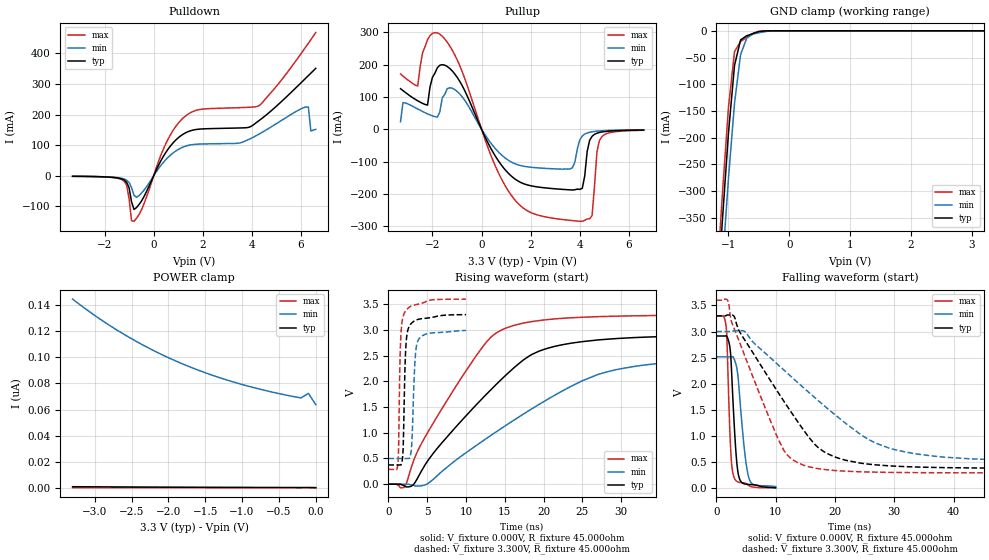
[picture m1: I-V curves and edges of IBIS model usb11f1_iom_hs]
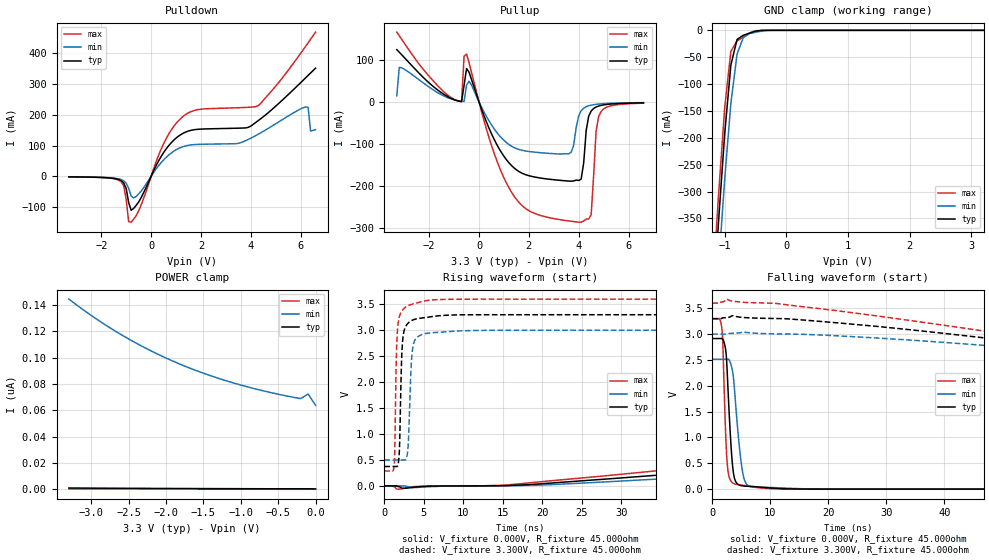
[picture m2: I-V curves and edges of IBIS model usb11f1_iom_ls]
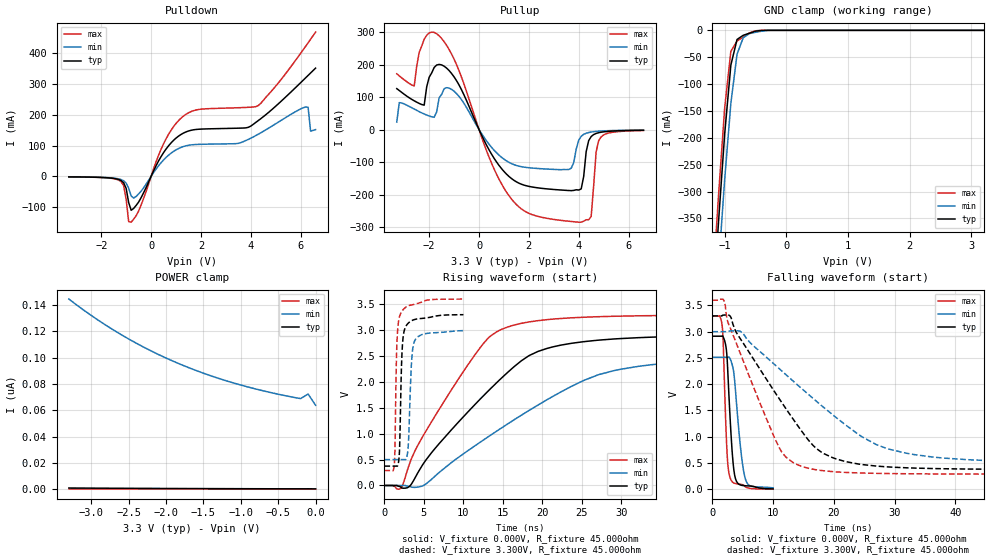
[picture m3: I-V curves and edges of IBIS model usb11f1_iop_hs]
[IBIS Ver]  4.0
[File Name]  lpc2939_lqfp208.ibs
[File Rev]  1.0
[Date]  Fri Feb 27 10:34:29 2009
[Source]  Package model is generic
[Notes]   IO models Rev 0.20 IBIS Model Design Automation Generation
[Copyright]  NXP Semiconductors 2009. All rights reserved.
[Disclaimer]
| NXP Semiconductors warrants and represents that the IBIS models
| identified herein are owned by NXP Semiconductors (NXP).  The
| models provided are not warranted as fully representing all of the
| operating characteristics and specifications of the semiconductor
| products to which the models relate.  Moreover, unless there is a
| signed, written agreement to the contrary, these models are furnished
| on an "as is" basis without support or warranty of any kind, either
| expressed or implied, regarding the use thereof, and NXP
| specifically disclaims all implied warranties of merchantability and
| fitness of the models for any purpose.
| NXP does not assume any liability arising out of the application
| or use of these IBIS models including infringement of patents and
| copyrights, nor does NXP convey any license under its patents and
| copyrights or the rights of others.
| NXP provides IBIS models as a service to our customers.  You and
| your company shall not distribute, convey, sell, or give these models
| to anyone else without receiving prior written permission from
| NXP.
[Component]   LPC23XX_LQFP208_01
[Manufacturer]  NXP
[Package]
|[Package Model]  LQFP208
|variable   typ   min   max
R_pkg   130.00m   123.00m   137.00m
L_pkg   8.30nH   7.50nH   9.20nH
C_pkg   1.00pF   0.80pF   1.30pF
| IMPORTANT NOTES:
| This model is valid for the following part types:
| LPC2939, LPC2930
| Signal names may be slightly different from the data
| sheet due to the 20 Char length limitation
[Pin]   signal_name   model_name   | comments
1 TDO bpats5thpept5v
2 P2_21 bpats5thpept5v
3 P0_24 bpats5thpept5v
4 P0_25 bpats5thpept5v
5 P0_26 bpats5thpept5v
6 P0_27 bpats5thpept5v
7 P0_28 bpats5thpept5v
8 P0_29 bpats5thpept5v
9 VDDE_10 POWER
10 P2_22 bpats5thpept5v
11 P2_23 bpats5thpept5v
12 P3_6 bpats5thpept5v
13 P3_7 bpats5thpept5v
14 P0_30 bpats5thpept5v
15 P0_31 bpats5thpept5v
16 P2_24 bpats5thpept5v
17 P2_25 bpats5thpept5v
18 GNDE_21 POWER
19 USB1_IOP usb11f1_iop_ls
20 USB1_IOM usb11f1_iom_ls
21 USB2_IOP usb11f1_iop_ls
22 USB2_IOM usb11f1_iom_ls
23 VDDE_26 POWER
24 VDD_27 POWER
25 GND_28 POWER
26 P1_31 bpats5thpept5v
27 GNDE_30 POWER
28 P4_0 bpats5thpept5v
29 P1_30 bpats5thpept5v
30 P5_0 bpats5thpept5v
31 P3_8 bpats5thpept5v
32 P3_9 bpats5thpept5v
33 P1_29 bpats5thpept5v
34 VDDE_37 POWER
35 P4_16 bpats5thpept5v
36 P1_28 bpats5thpept5v
37 P2_26 bpats5thpept5v
38 P4_8 bpats5thpept5v
39 GNDE_42 POWER
40 P2_27 bpats5thpept5v
41 P5_8 bpats5thpept5v
42 P1_27 bpats5thpept5v
43 P1_26 bpats5thpept5v
44 P4_20 bpats5thpept5v
45 VDDE_48 POWER
46 P1_25 bpats5thpept5v
47 GND_50 POWER
48 VDD_51 POWER
49 P1_24 bpats5thpept5v
50 P1_23 bpats5thpept5v
51 P1_22 bpats5thpept5v
52 TMS bpats5thpept5v
53 TCK bpats5thpept5v
54 P1_21 bpats5thpept5v
55 P1_20 bpats5thpept5v
56 P1_19 bpats5thpept5v
57 P1_18 bpats5thpept5v
58 P1_17 bpats5thpept5v
59 GNDE_62 POWER
60 P4_4 bpats5thpept5v
61 P1_16 bpats5thpept5v
62 P5_4 bpats5thpept5v
63 P2_0 bpats5thpept5v
64 P4_12 bpats5thpept5v
65 P2_1 bpats5thpept5v
66 P5_12 bpats5thpept5v
67 VDDE_70 POWER
68 P4_1 bpats5thpept5v
69 P3_10 bpats5thpept5v
70 GND_73 POWER
71 VDD_74 POWER
72 P5_1 bpats5thpept5v
73 P3_11 bpats5thpept5v
74 P4_17 bpats5thpept5v
75 P1_15 bpats5thpept5v
76 P4_9 bpats5thpept5v
77 GNDE_80 POWER
78 P5_9 bpats5thpept5v
79 P1_14 bpats5thpept5v
80 P4_21 bpats5thpept5v
81 P1_13 bpats5thpept5v
82 P4_5 bpats5thpept5v
83 P1_12 bpats5thpept5v
84 P5_5 bpats5thpept5v
85 VDDE_88 POWER
86 P2_2 bpats5thpept5v
87 P2_3 bpats5thpept5v
88 P1_11 bpats5thpept5v
89 P1_10 bpats5thpept5v
90 P3_12 bpats5thpept5v
91 GND_94 POWER
92 VDD_95 POWER
93 P3_13 bpats5thpept5v
94 P2_4 bpats5thpept5v
95 P2_5 bpats5thpept5v
96 P1_9 bpats5thpept5v
97 GNDE_100 POWER
98 P1_8 bpats5thpept5v
99 P1_7 bpats5thpept5v
100 P1_6 bpats5thpept5v
101 P2_6 bpats5thpept5v
102 P1_5 bpats5thpept5v
103 P1_4 bpats5thpept5v
104 TRSTN bpats5thpept5v
105 RSTN bpats5thpept5v
106 VSSA_OSC_1 POWER
107 XOUT_OSC NC
108 XIN_OSC NC
109 VDDA_OSC POWER
110 VSSA_PLL_1 POWER
111 P2_7 bpats5thpept5v
112 P3_14 bpats5thpept5v
113 P3_15 bpats5thpept5v
114 VDDE_119 POWER
115 P2_8 bpats5thpept5v
116 P2_9 bpats5thpept5v
117 P1_3 bpats5thpept5v
118 P1_2 bpats5thpept5v
119 P1_1 bpats5thpept5v
120 GND_125 POWER
121 VDD_127 POWER
122 P1_0 bpats5thpept5v
123 P2_10 bpats5thpept5v
124 P2_11 bpats5thpept5v
125 P0_0 bpats5thpept5v
126 GNDE_134 POWER
127 P4_13 bpats5thpept5v
128 P0_1 bpats5thpept5v
129 P5_13 bpats5thpept5v
130 P0_2 bpats5thpept5v
131 P4_2 bpats5thpept5v
132 VDDE_141 POWER
133 P5_2 bpats5thpept5v
134 P0_3 bpats5thpept5v
135 P4_18 bpats5thpept5v
136 P3_0 bpats5thpept5v
137 P4_10 bpats5thpept5v
138 P3_1 bpats5thpept5v
139 P5_10 bpats5thpept5v
140 P2_12 bpats5thpept5v
141 VDD_150 POWER
142 GND_151 POWER
143 P4_22 bpats5thpept5v
144 GNDE_153 POWER
145 P2_13 bpats5thpept5v
146 P4_6 bpats5thpept5v
147 P0_4 bpats5thpept5v
148 P5_6 bpats5thpept5v
149 P4_14 bpats5thpept5v
150 P0_5 bpats5thpept5v
151 P5_14 bpats5thpept5v
152 VDDE_161 POWER
153 P0_6 bpats5thpept5v
154 P0_7 bpats5thpept5v
155 A3V3 POWER
156 JTAGSEL bpats5thpept5v
157 A5V POWER
158 VREFP NC
159 VREFN NC
160 P0_8 bpats5thpept5v
161 P0_9 bpats5thpept5v
162 P0_10 bpats5thpept5v
163 P0_11 bpats5thpept5v
164 P2_14 bpats5thpept5v
165 P2_15 bpats5thpept5v
166 P3_2 bpats5thpept5v
167 VDD_176 POWER
168 GND_177 POWER
169 GNDE_178 POWER
170 P4_3 bpats5thpept5v
171 P3_3 bpats5thpept5v
172 P5_3 bpats5thpept5v
173 P0_12 bpats5thpept5v
174 P4_19 bpats5thpept5v
175 P0_13 bpats5thpept5v
176 VDDE_185 POWER
177 P4_11 bpats5thpept5v
178 P0_14 bpats5thpept5v
179 P5_11 bpats5thpept5v
180 P0_15 bpats5thpept5v
181 P4_23 bpats5thpept5v
182 P0_16 bpats5thpept5v
183 P4_7 bpats5thpept5v
184 GNDE_193 POWER
185 P5_7 bpats5thpept5v
186 P0_17 bpats5thpept5v
187 P4_15 bpats5thpept5v
188 P5_15 bpats5thpept5v
189 VDD_198 POWER
190 GND_199 POWER
191 P2_16 bpats5thpept5v
192 P2_17 bpats5thpept5v
193 VDDE_202 POWER
194 P0_18 bpats5thpept5v
195 P0_19 bpats5thpept5v
196 P3_4 bpats5thpept5v
197 P3_5 bpats5thpept5v
198 P2_18 bpats5thpept5v
199 P2_19 bpats5thpept5v
200 P0_20 bpats5thpept5v
201 P0_21 bpats5thpept5v
202 P0_22 bpats5thpept5v
203 GNDE_212 POWER
204 P0_23 bpats5thpept5v
205 P2_20 bpats5thpept5v
206 VDD_215 POWER
207 GND_216 POWER
208 TDI bpats5thpept5v
[Model Selector] bpats5thpept5v
bpats5thpept5v_p   Plain input Mode (p1=0, p2=1)
bpats5thpept5v_pd   Pull Down Mode   (p1=0, p2=0)
bpats5thpept5v_pu   Pull up   Mode   (p1=1, p2=1)
bpats5thpept5v_r   Repeater  Mode   (p1=1, p2=0)
[Model Selector] bpts5ptpht5v
bpts5ptpht5v_p_sh   Plain input Mode (p1=0, p2=1)
bpts5ptpht5v_p_sl   Plain input Mode (p1=0, p2=1)
bpts5ptpht5v_pd_sh   Pull Down Mode (p1=1, p2=1)
bpts5ptpht5v_pd_sl   Pull Down Mode (p1=1, p2=1)
bpts5ptpht5v_pu_sh   Pull Up Mode (p1=0, p2=0)
bpts5ptpht5v_pu_sl   Pull Up Mode (p1=0, p2=0)
bpts5ptpht5v_r_sh   Repeater Mode (p1=1, p2=0)
bpts5ptpht5v_r_sl   Repeater Mode (p1=1, p2=0)
| Models and submodels in the file (16): usb11f1_iom_hs (I/O), usb11f1_iom_ls (I/O), usb11f1_iop_hs (I/O), usb11f1_iop_ls (I/O), bpats5thpept5v_p (I/O), bpats5thpept5v_pd (I/O), bpats5thpept5v_pu (I/O), bpats5thpept5v_r (I/O), bpts5ptpht5v_p_sh (I/O), bpts5ptpht5v_p_sl (I/O), bpts5ptpht5v_pd_sh (I/O), bpts5ptpht5v_pd_sl (I/O), bpts5ptpht5v_pu_sh (I/O), bpts5ptpht5v_pu_sl (I/O), bpts5ptpht5v_r_sh (I/O), bpts5ptpht5v_r_sl (I/O)
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| usb11f1
|   Universal Serial Bus Pad
|   Revision 1.1 Specification
|   Programmable Single Ended Core Input
|   Forced Single Ended Low
|   Switchable between
|   - high speed output mode
|   - low speed output mode
|   - low/high speed input mode
| |   Rev 0.20 IBIS Model Design Automation Generation   |
| |   N O N - S I L I C O N   C O R R E L A T E D   |
| |   This IBIS [Model] is pre-Beta tactical support   |
| |  Note: this IBIS [Model] contains clamp curves generated   |
| |   through simulation which should not be relied upon   |
| Pccmos14 hliolib_nlm 4.0
|   0.18 um 3.3V pad library
|   six level metal
|   dual oxide
|   single threshold voltage
|   nominal line mixed supply
|   parasitic extracted netlists
| Process block c14
| High Speed Output Mode
[Model]   usb11f1_iom_hs | of usb11f1
Model_type   I/O
Polarity   Non-Inverting
Enable   Active-Low
|  Reciever Thresholds
Vinl   = 0.8V
Vinh   = 2.0V
| AC Test Load Conditions
Vref   = 0
Cref   = 0
Rref   = 1000000000
Vmeas   = 1.65
| [Process Range]   typical   min   max
| C_comp edge width   400.000ps   400.000ps   400.000ps
| C_comp Tstrobe   40.000fs   40.000fs   40.000fs
C_comp   3.752pF   3.496pF   4.045pF
[Temperature Range]   25   125   -40
[Voltage Range]   3.30V   3.00V   3.60V
[GND Clamp Reference]   0.00V   0.00V   0.00V
[Pulldown Reference]   0.00V   0.00V   0.00V
[POWER Clamp Reference]   3.30V   3.00V   3.60V
[Pullup Reference]   3.30V   3.00V   3.60V
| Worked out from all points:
|   slope of the pulldown table from 0 to 0.495 V, typ, clamps not added: 6.48 ohm
|   slope of the pullup table from 0 to 0.495 V, typ, clamps not added: 6.61 ohm
|   GND clamp passes 1 mA (typ) near -0.46 V on its own axis
|   rising waveform, V_fixture 0.000V, R_fixture 45.000ohm: 20-80 % time 11ns typ, 15.9ns min, 8.17ns max; typ from 0 V to 2.91 V
|   falling waveform, V_fixture 0.000V, R_fixture 45.000ohm: 20-80 % time 845ps typ, 1.21ns min, 607ps max; typ from 2.91 V to 0.006 V
|   rising waveform, V_fixture 3.300V, R_fixture 45.000ohm: 20-80 % time 320ps typ, 399ps min, 287ps max; typ from 0.374 V to 3.3 V
|   falling waveform, V_fixture 3.300V, R_fixture 45.000ohm: 20-80 % time 10.2ns typ, 15.5ns min, 6.95ns max; typ from 3.3 V to 0.374 V
[GND Clamp]
| ref voltage   0.00V   0.00V   0.00V
|   Voltage   I(typ)   I(min)   I(max)
-3.3V     -4.618A    -4.67A     -4.591A
-1.2V     -533.4mA   -616mA     -486.2mA
-1.1V     -356.1mA   -441.1mA   -306.9mA
-1V       -192.1mA   -277.1mA   -143.8mA
-900mV    -64.59mA   -135.6mA   -38.91mA
-800mV    -17.04mA   -44.51mA   -19.95mA
-700mV    -9.237mA   -13.86mA   -12.52mA
-600mV    -5.456mA   -6.064mA   -4.789mA
-500mV    -1.495mA   -3.666mA   -840.2uA
-300mV    -6.625uA   -179.7uA   -408.9nA
3.2V      293.2pA    68.89nA    105.6pA
[Power Clamp]   | Vtable = Vcc - Vpad
| ref voltage   3.30V   3.00V   3.60V
|   Voltage   I(typ)   I(min)   I(max)
-3.3V     1.005nA    144.5nA    354.7pA
-3V       911.2pA    132nA      335.1pA
-2.6V     800.8pA    117.4nA    309pA
-2.3V     727.5pA    108nA      289.6pA
-1.9V     640.7pA    97.15nA    263.8pA
-1.6V     582.9pA    90.25nA    244.5pA
-1.3V     530.6pA    84.3nA     225.3pA
-1V       483pA      79.18nA    206.1pA
-700mV    439.6pA    74.79nA    187pA
-200mV    377.6pA    68.89nA    155pA
-100mV    416.5pA    72.39nA    142.6pA
0V        319.1pA    63.83nA    125.6pA
[Pulldown]
| ref voltage   0.00V   0.00V   0.00V
|   Voltage   I(typ)   I(min)   I(max)
-3.3V     -1.652mA   -1.454mA   -1.796mA
-1.2V     -13.92mA   -10.45mA   -17.73mA
-1.1V     -21.12mA   -14.45mA   -30.61mA
-900mV    -85.23mA   -38.63mA   -146.6mA
-800mV    -110mA     -63.62mA   -148.7mA
500mV     77.03mA    53.28mA    105.7mA
1.1V      130.5mA    90.36mA    180.9mA
4.3V      181mA      136.8mA    229.8mA
6.2V      319.7mA    225.1mA    421.9mA
6.3V      327.6mA    224.1mA    433.3mA
6.4V      335.5mA    146.8mA    444.9mA
6.6V      351.2mA    151.8mA    468.2mA
[Pullup]   | Vtable = Vcc - Vpad
| ref voltage   3.30V   3.00V   3.60V
|   Voltage   I(typ)   I(min)   I(max)
-3.3V     125.8mA    23.2mA     171.5mA
-2.6V     88.3mA     62.98mA    134mA
-2.2V     74.98mA    47.7mA     277.9mA
-1.6V     200.3mA    97.67mA    288.3mA
-1V       161.8mA    117.7mA    216.4mA
900mV     -120mA     -85.3mA    -166.8mA
2.5V      -180.9mA   -120.7mA   -269.8mA
3.7V      -188.1mA   -119.1mA   -283mA
4.1V      -182.9mA   -20.96mA   -285.2mA
4.4V      -34.22mA   -9.287mA   -277.5mA
4.8V      -9.883mA   -5.195mA   -34.66mA
6.6V      -2.365mA   -1.804mA   -3.161mA
[Ramp]
R_load   = 60.000ohm
|   dV/dt(typ)   dV/dt(min)   dV/dt(max)
dV/dt_r   803.394mV/4.105ns   370.492mV/2.885ns   1.331V/4.905ns
dV/dt_f   843.371mV/4.620ns   360.067mV/3.240ns   1.540V/5.255ns
[Rising Waveform]  | cubic spline decimation from 16001 points
V_fixture   = 0.000V
R_fixture   = 45.000ohm
|   Time   V(typ)   V(min)   V(max)
0s        443.9pV    34.48nV    250.2pV
2.05ns    -28.68mV   9.864uV    -55.51mV
3.165ns   -16.71mV   -18.22mV   419.1mV
5.14ns    468.7mV    16.86mV    1.024V
12.03ns   1.653V     825.1mV    2.643V
16.32ns   2.281V     1.258V     3.093V
21.57ns   2.684V     1.741V     3.215V
26.99ns   2.804V     2.132V     3.257V
32.92ns   2.858V     2.315V     3.276V
80ns      2.912V     2.506V     3.295V
[Falling Waveform]  | cubic spline decimation from 2001 points
V_fixture   = 0.000V
R_fixture   = 45.000ohm
|   Time   V(typ)   V(min)   V(max)
0s        2.914V     2.514V     3.296V
1.65ns    2.919V     2.514V     3.102V
1.79ns    2.905V     2.514V     2.86V
2.415ns   2.567V     2.514V     760.7mV
2.935ns   1.397V     2.492V     222.4mV
3.365ns   607.8mV    2.348V     134.4mV
3.78ns    227.5mV    1.985V     109.9mV
4.655ns   81.21mV    824.9mV    94.37mV
5.45ns    66.93mV    210.5mV    47.53mV
10ns      6.197mV    27.24mV    1.84mV
[Rising Waveform]  | cubic spline decimation from 2001 points
V_fixture   = 3.300V
V_fixture_min = 3.000V
V_fixture_max = 3.600V
R_fixture   = 45.000ohm
|   Time   V(typ)   V(min)   V(max)
0s        373.7mV    499.4mV    287.7mV
1.215ns   373.7mV    499.4mV    375.2mV
1.575ns   374.2mV    499.5mV    2.78V
1.87ns    595mV      499.5mV    3.244V
2.065ns   1.779V     499.5mV    3.327V
2.355ns   2.862V     499.5mV    3.393V
2.96ns    3.126V     677.4mV    3.465V
3.43ns    3.18V      2.396V     3.486V
3.84ns    3.205V     2.798V     3.499V
10ns      3.296V     2.989V     3.598V
[Falling Waveform]  | cubic spline decimation from 16001 points
V_fixture   = 3.300V
V_fixture_min = 3.000V
V_fixture_max = 3.600V
R_fixture   = 45.000ohm
|   Time   V(typ)   V(min)   V(max)
0s        3.3V       3V         3.6V
1.96ns    3.316V     3V         3.585V
2.955ns   3.297V     3.013V     3.074V
4.81ns    2.836V     3V         2.532V
11.41ns   1.661V     2.26V      717.5mV
14.73ns   1.108V     1.92V      436.6mV
20.49ns   574.7mV    1.36V      330.4mV
25.63ns   457.1mV    931.8mV    306.2mV
31.99ns   408.5mV    686.3mV    295.4mV
80ns      374.5mV    503.6mV    287.9mV
| usb11f1
|   Universal Serial Bus Pad
|   Revision 1.1 Specification
|   Programmable Single Ended Core Input
|   Forced Single Ended Low
|   Switchable between
|   - high speed output mode
|   - low speed output mode
|   - low/high speed input mode
| |   Rev 0.20 IBIS Model Design Automation Generation   |
| |   N O N - S I L I C O N   C O R R E L A T E D   |
| |   This IBIS [Model] is pre-Beta tactical support   |
| |  Note: this IBIS [Model] contains clamp curves generated   |
| |   through simulation which should not be relied upon   |
| Pccmos14 hliolib_nlm 4.0
|   0.18 um 3.3V pad library
|   six level metal
|   dual oxide
|   single threshold voltage
|   nominal line mixed supply
|   parasitic extracted netlists
| Process block c14
| Low Speed Output Mode
[Model]   usb11f1_iom_ls | of usb11f1
Model_type   I/O
Polarity   Non-Inverting
Enable   Active-Low
|  Reciever Thresholds
Vinl   = 0.8V
Vinh   = 2.0V
| AC Test Load Conditions
Vref   = 0
Cref   = 0
Rref   = 1000000000
Vmeas   = 1.65
| [Process Range]   typical   min   max
| C_comp edge width   400.000ps   400.000ps   400.000ps
| C_comp Tstrobe   40.000fs   40.000fs   40.000fs
C_comp   3.752pF   3.496pF   4.045pF
[Temperature Range]   25   125   -40
[Voltage Range]   3.30V   3.00V   3.60V
[GND Clamp Reference]   0.00V   0.00V   0.00V
[Pulldown Reference]   0.00V   0.00V   0.00V
[POWER Clamp Reference]   3.30V   3.00V   3.60V
[Pullup Reference]   3.30V   3.00V   3.60V
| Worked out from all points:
|   slope of the pulldown table from 0 to 0.495 V, typ, clamps not added: 6.48 ohm
|   slope of the pullup table from 0 to 0.495 V, typ, clamps not added: 6.61 ohm
|   GND clamp passes 1 mA (typ) near -0.46 V on its own axis
|   rising waveform, V_fixture 0.000V, R_fixture 45.000ohm: 20-80 % time 151ns typ, 180ns min, 132ns max; typ from 0 V to 2.91 V
|   falling waveform, V_fixture 0.000V, R_fixture 45.000ohm: 20-80 % time 850ps typ, 1.23ns min, 609ps max; typ from 2.91 V to 0 V
|   rising waveform, V_fixture 3.300V, R_fixture 45.000ohm: 20-80 % time 318ps typ, 398ps min, 284ps max; typ from 0.374 V to 3.3 V
|   falling waveform, V_fixture 3.300V, R_fixture 45.000ohm: 20-80 % time 156ns typ, 194ns min, 133ns max; typ from 3.3 V to 0.38 V
[GND Clamp]
| ref voltage   0.00V   0.00V   0.00V
|   Voltage   I(typ)   I(min)   I(max)
-3.3V     -4.618A    -4.67A     -4.591A
-1.2V     -533.4mA   -616mA     -486.2mA
-1.1V     -356.1mA   -441.1mA   -306.9mA
-1V       -192.1mA   -277.1mA   -143.8mA
-900mV    -64.59mA   -135.6mA   -38.91mA
-800mV    -17.04mA   -44.51mA   -19.95mA
-700mV    -9.237mA   -13.86mA   -12.52mA
-600mV    -5.456mA   -6.064mA   -4.789mA
-500mV    -1.495mA   -3.666mA   -840.2uA
-300mV    -6.625uA   -179.7uA   -408.9nA
3.2V      293.2pA    68.89nA    105.6pA
[Power Clamp]   | Vtable = Vcc - Vpad
| ref voltage   3.30V   3.00V   3.60V
|   Voltage   I(typ)   I(min)   I(max)
-3.3V     1.005nA    144.5nA    354.7pA
-3V       911.2pA    132nA      335.1pA
-2.6V     800.8pA    117.4nA    309pA
-2.3V     727.5pA    108nA      289.6pA
-1.9V     640.7pA    97.15nA    263.8pA
-1.6V     582.9pA    90.25nA    244.5pA
-1.3V     530.6pA    84.3nA     225.3pA
-1V       483pA      79.18nA    206.1pA
-700mV    439.6pA    74.79nA    187pA
-200mV    377.6pA    68.89nA    155pA
-100mV    416.5pA    72.39nA    142.6pA
0V        319.1pA    63.83nA    125.6pA
[Pulldown]
| ref voltage   0.00V   0.00V   0.00V
|   Voltage   I(typ)   I(min)   I(max)
-3.3V     -1.652mA   -1.454mA   -1.796mA
-1.2V     -13.92mA   -10.45mA   -17.73mA
-1.1V     -21.12mA   -14.45mA   -30.61mA
-900mV    -85.23mA   -38.63mA   -146.6mA
-800mV    -110mA     -63.62mA   -148.7mA
500mV     77.03mA    53.28mA    105.7mA
1.1V      130.5mA    90.36mA    180.9mA
4.3V      181mA      136.8mA    229.8mA
6.2V      319.7mA    225.1mA    421.9mA
6.3V      327.6mA    224.1mA    433.3mA
6.4V      335.5mA    146.8mA    444.9mA
6.6V      351.2mA    151.8mA    468.2mA
[Pullup]   | Vtable = Vcc - Vpad
| ref voltage   3.30V   3.00V   3.60V
|   Voltage   I(typ)   I(min)   I(max)
-3.3V     123.9mA    14.28mA    165.4mA
-3.2V     117.8mA    81.84mA    156.7mA
-800mV    1.807mA    2.206mA    1.368mA
-500mV    79.1mA     39.57mA    113.5mA
1V        -129mA     -91.21mA   -180.1mA
2.5V      -180.9mA   -120.7mA   -269.8mA
3.7V      -188.1mA   -119.1mA   -283mA
4.1V      -182.9mA   -20.96mA   -285.2mA
4.4V      -34.22mA   -9.287mA   -277.5mA
4.5V      -21.68mA   -7.778mA   -267.6mA
4.8V      -9.883mA   -5.195mA   -34.66mA
6.6V      -2.365mA   -1.804mA   -3.161mA
[Ramp]
R_load   = 60.000ohm
|   dV/dt(typ)   dV/dt(min)   dV/dt(max)
dV/dt_r   621.133mV/49.000ns   449.857mV/47.650ns   797.798mV/50.350ns
dV/dt_f   625.100mV/49.850ns   419.096mV/47.300ns   836.278mV/52.000ns
[Rising Waveform]  | cubic spline decimation from 16001 points
V_fixture   = 0.000V
R_fixture   = 45.000ohm
|   Time   V(typ)   V(min)   V(max)
0s        443.9pV    34.49nV    250.2pV
1.75ns    -12.65mV   2.275uV    -62.94mV
15.6ns    5.793mV    2.484mV    18.34mV
130.2ns   1.408V     1.033V     1.795V
182.8ns   2.006V     1.49V      2.541V
215.3ns   2.324V     1.742V     2.891V
240.8ns   2.515V     1.918V     3.033V
308.5ns   2.738V     2.227V     3.184V
402.4ns   2.838V     2.384V     3.248V
800ns     2.907V     2.501V     3.292V
[Falling Waveform]  | cubic spline decimation from 2001 points
V_fixture   = 0.000V
R_fixture   = 45.000ohm
|   Time   V(typ)   V(min)   V(max)
0s        2.914V     2.514V     3.296V
1.65ns    2.918V     2.514V     3.099V
1.8ns     2.902V     2.514V     2.824V
2.25ns    2.726V     2.514V     1.203V
2.75ns    1.81V      2.518V     313.5mV
3.35ns    628.5mV    2.352V     134.1mV
3.85ns    197.5mV    1.878V     99.95mV
5.3ns     62.15mV    280.7mV    75.31mV
6.75ns    52.95mV    48.63mV    46.78mV
100ns     89.79uV    122.2uV    67.53uV
[Rising Waveform]  | cubic spline decimation from 2001 points
V_fixture   = 3.300V
V_fixture_min = 3.000V
V_fixture_max = 3.600V
R_fixture   = 45.000ohm
|   Time   V(typ)   V(min)   V(max)
0s        373.7mV    499.4mV    287.7mV
1.25ns    373.7mV    499.5mV    440.2mV
1.55ns    374.8mV    499.5mV    2.698V
1.85ns    558.6mV    499.5mV    3.237V
2.15ns    2.321V     499.5mV    3.356V
2.4ns     2.919V     499.6mV    3.406V
3ns       3.136V     762.4mV    3.473V
3.6ns     3.197V     2.674V     3.505V
4.85ns    3.237V     2.922V     3.556V
100ns     3.3V       3V         3.6V
[Falling Waveform]  | cubic spline decimation from 16001 points
V_fixture   = 3.300V
V_fixture_min = 3.000V
V_fixture_max = 3.600V
R_fixture   = 45.000ohm
|   Time   V(typ)   V(min)   V(max)
0s        3.3V       3V         3.6V
2.45ns    3.319V     3V         3.678V
28.5ns    3.148V     2.924V     3.35V
114.5ns   2.081V     2.172V     1.981V
188.3ns   1.259V     1.566V     937.8mV
232.7ns   858.8mV    1.248V     557.2mV
289.8ns   591.2mV    921.5mV    405.8mV
389.9ns   453.5mV    659.5mV    332.3mV
557.6ns   398mV      548.8mV    301.5mV
800ns     380mV      513mV      291.2mV
| usb11f1
|   Universal Serial Bus Pad
|   Revision 1.1 Specification
|   Programmable Single Ended Core Input
|   Forced Single Ended Low
|   Switchable between
|   - high speed output mode
|   - low speed output mode
|   - low/high speed input mode
| |   Rev 0.20 IBIS Model Design Automation Generation   |
| |   N O N - S I L I C O N   C O R R E L A T E D   |
| |   This IBIS [Model] is pre-Beta tactical support   |
| |  Note: this IBIS [Model] contains clamp curves generated   |
| |   through simulation which should not be relied upon   |
| Pccmos14 hliolib_nlm 4.0
|   0.18 um 3.3V pad library
|   six level metal
|   dual oxide
|   single threshold voltage
|   nominal line mixed supply
|   parasitic extracted netlists
| Process block c14
| High Speed Output Mode
[Model]   usb11f1_iop_hs | of usb11f1
Model_type   I/O
Polarity   Non-Inverting
Enable   Active-Low
|  Reciever Thresholds
Vinl   = 0.8V
Vinh   = 2.0V
| AC Test Load Conditions
Vref   = 0
Cref   = 0
Rref   = 1000000000
Vmeas   = 1.65
| [Process Range]   typical   min   max
| C_comp edge width   400.000ps   400.000ps   400.000ps
| C_comp Tstrobe   40.000fs   40.000fs   40.000fs
C_comp   3.752pF   3.496pF   4.045pF
[Temperature Range]   25   125   -40
[Voltage Range]   3.30V   3.00V   3.60V
[GND Clamp Reference]   0.00V   0.00V   0.00V
[Pulldown Reference]   0.00V   0.00V   0.00V
[POWER Clamp Reference]   3.30V   3.00V   3.60V
[Pullup Reference]   3.30V   3.00V   3.60V
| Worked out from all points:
|   slope of the pulldown table from 0 to 0.495 V, typ, clamps not added: 6.48 ohm
|   slope of the pullup table from 0 to 0.495 V, typ, clamps not added: 6.61 ohm
|   GND clamp passes 1 mA (typ) near -0.46 V on its own axis
|   rising waveform, V_fixture 0.000V, R_fixture 45.000ohm: 20-80 % time 11ns typ, 15.9ns min, 8.17ns max; typ from 0 V to 2.91 V
|   falling waveform, V_fixture 0.000V, R_fixture 45.000ohm: 20-80 % time 847ps typ, 1.21ns min, 606ps max; typ from 2.91 V to 0.006 V
|   rising waveform, V_fixture 3.300V, R_fixture 45.000ohm: 20-80 % time 321ps typ, 402ps min, 285ps max; typ from 0.374 V to 3.3 V
|   falling waveform, V_fixture 3.300V, R_fixture 45.000ohm: 20-80 % time 10.2ns typ, 15.5ns min, 6.95ns max; typ from 3.3 V to 0.374 V
[GND Clamp]
| ref voltage   0.00V   0.00V   0.00V
|   Voltage   I(typ)   I(min)   I(max)
-3.3V     -4.618A    -4.67A     -4.591A
-1.2V     -533.4mA   -616mA     -486.2mA
-1.1V     -356.1mA   -441.1mA   -306.9mA
-1V       -192.1mA   -277.1mA   -143.8mA
-900mV    -64.59mA   -135.6mA   -38.91mA
-800mV    -17.04mA   -44.51mA   -19.95mA
-700mV    -9.237mA   -13.86mA   -12.52mA
-600mV    -5.456mA   -6.064mA   -4.789mA
-500mV    -1.495mA   -3.666mA   -840.2uA
-300mV    -6.625uA   -179.7uA   -408.9nA
3.2V      293.2pA    68.89nA    105.6pA
[Power Clamp]   | Vtable = Vcc - Vpad
| ref voltage   3.30V   3.00V   3.60V
|   Voltage   I(typ)   I(min)   I(max)
-3.3V     1.005nA    144.5nA    354.7pA
-3V       911.2pA    132nA      335.1pA
-2.6V     800.8pA    117.4nA    309pA
-2.3V     727.5pA    108nA      289.6pA
-1.9V     640.7pA    97.15nA    263.8pA
-1.6V     582.9pA    90.25nA    244.5pA
-1.3V     530.6pA    84.3nA     225.3pA
-1V       483pA      79.18nA    206.1pA
-700mV    439.6pA    74.79nA    187pA
-200mV    377.6pA    68.89nA    155pA
-100mV    416.5pA    72.39nA    142.6pA
0V        319.1pA    63.83nA    125.6pA
[Pulldown]
| ref voltage   0.00V   0.00V   0.00V
|   Voltage   I(typ)   I(min)   I(max)
-3.3V     -1.652mA   -1.454mA   -1.796mA
-1.2V     -13.92mA   -10.45mA   -17.73mA
-1.1V     -21.12mA   -14.45mA   -30.61mA
-900mV    -85.23mA   -38.63mA   -146.6mA
-800mV    -110mA     -63.62mA   -148.7mA
500mV     77.03mA    53.28mA    105.7mA
1.1V      130.5mA    90.36mA    180.9mA
4.3V      181mA      136.8mA    229.8mA
6.2V      319.7mA    225.1mA    421.9mA
6.3V      327.6mA    224.1mA    433.3mA
6.4V      335.5mA    146.8mA    444.9mA
6.6V      351.2mA    151.8mA    468.2mA
[Pullup]   | Vtable = Vcc - Vpad
| ref voltage   3.30V   3.00V   3.60V
|   Voltage   I(typ)   I(min)   I(max)
-3.3V     125.8mA    23.2mA     171.5mA
-2.6V     88.3mA     62.98mA    134mA
-2.2V     74.98mA    47.7mA     277.9mA
-1.6V     200.3mA    97.67mA    288.3mA
-1V       161.8mA    117.7mA    216.4mA
900mV     -120mA     -85.3mA    -166.8mA
2.5V      -180.9mA   -120.7mA   -269.8mA
3.7V      -188.1mA   -119.1mA   -283mA
4.1V      -182.9mA   -20.96mA   -285.2mA
4.4V      -34.22mA   -9.287mA   -277.5mA
4.8V      -9.883mA   -5.195mA   -34.66mA
6.6V      -2.365mA   -1.804mA   -3.161mA
[Ramp]
R_load   = 60.000ohm
|   dV/dt(typ)   dV/dt(min)   dV/dt(max)
dV/dt_r   802.872mV/4.105ns   370.430mV/2.890ns   1.330V/4.895ns
dV/dt_f   847.049mV/4.645ns   363.155mV/3.270ns   1.544V/5.270ns
[Rising Waveform]  | cubic spline decimation from 16001 points
V_fixture   = 0.000V
R_fixture   = 45.000ohm
|   Time   V(typ)   V(min)   V(max)
0s        443.9pV    34.48nV    250.2pV
2.065ns   -29.58mV   -1.03uV    -55.15mV
3.17ns    -16.87mV   -18.22mV   416.1mV
5.21ns    482.5mV    23.6mV     1.039V
12.08ns   1.661V     830.7mV    2.652V
16.39ns   2.289V     1.265V     3.095V
21.33ns   2.675V     1.719V     3.211V
26.95ns   2.803V     2.13V      3.257V
32.18ns   2.853V     2.3V       3.275V
80ns      2.912V     2.506V     3.295V
[Falling Waveform]  | cubic spline decimation from 2001 points
V_fixture   = 0.000V
R_fixture   = 45.000ohm
|   Time   V(typ)   V(min)   V(max)
0s        2.914V     2.514V     3.296V
1.64ns    2.92V      2.514V     3.086V
1.765ns   2.904V     2.514V     2.86V
2.38ns    2.57V      2.514V     783.4mV
2.935ns   1.326V     2.481V     213.7mV
3.41ns    505.1mV    2.301V     127.8mV
3.77ns    217.1mV    1.933V     109.5mV
4.66ns    79.74mV    768.8mV    93.98mV
5.445ns   66.7mV     193.7mV    45.74mV
10ns      6.095mV    26.73mV    1.823mV
[Rising Waveform]  | cubic spline decimation from 2001 points
V_fixture   = 3.300V
V_fixture_min = 3.000V
V_fixture_max = 3.600V
R_fixture   = 45.000ohm
|   Time   V(typ)   V(min)   V(max)
0s        373.7mV    499.4mV    287.7mV
1.245ns   373.7mV    499.4mV    398.8mV
1.58ns    374.4mV    499.5mV    2.748V
1.88ns    599.6mV    499.5mV    3.241V
2.075ns   1.793V     499.5mV    3.326V
2.365ns   2.864V     499.5mV    3.393V
2.965ns   3.125V     677.1mV    3.464V
3.435ns   3.18V      2.395V     3.485V
3.815ns   3.203V     2.788V     3.498V
10ns      3.296V     2.989V     3.598V
[Falling Waveform]  | cubic spline decimation from 16001 points
V_fixture   = 3.300V
V_fixture_min = 3.000V
V_fixture_max = 3.600V
R_fixture   = 45.000ohm
|   Time   V(typ)   V(min)   V(max)
0s        3.3V       3V         3.6V
1.905ns   3.316V     3V         3.592V
2.51ns    3.319V     3V         3.198V
5.015ns   2.793V     2.974V     2.463V
11.14ns   1.702V     2.283V     764.9mV
14.69ns   1.108V     1.918V     436.9mV
20.36ns   578.2mV    1.367V     331.2mV
27ns      441.4mV    850.1mV    302.8mV
32.03ns   408.2mV    684.4mV    295.3mV
80ns      374.5mV    503.6mV    287.9mV
